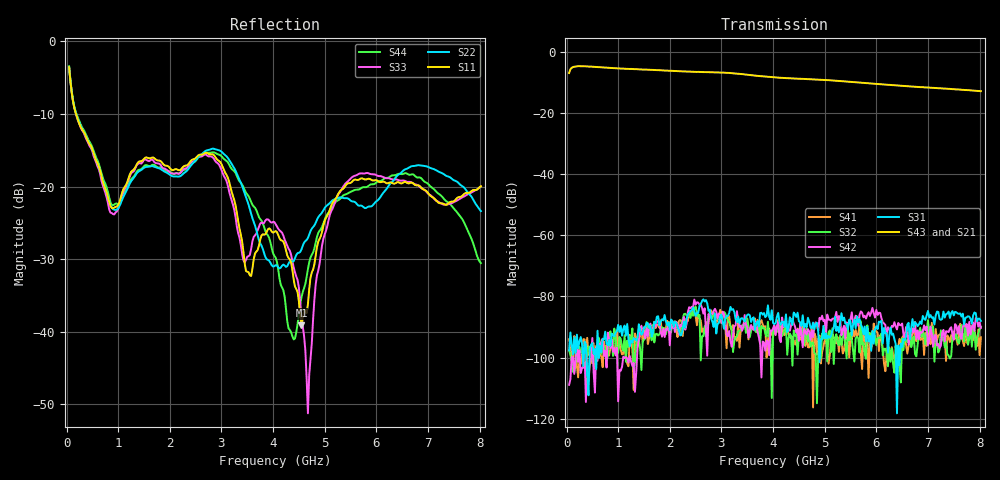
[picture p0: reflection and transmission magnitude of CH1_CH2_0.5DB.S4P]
!Agilent Technologies,E5071C,MY46316741,A.11.02
!Date: Thu May 28 14:25:22 2026
!Data & Calibration Information:
!1:CH1 INPUT 2:CH1 OUTPUT 3:CH2 INPUT 4:CH2 OUTPUT
!Freq	S11:SOLT4(ON)	S12:SOLT4(ON)	S13:SOLT4(ON)	S14:SOLT4(ON)
!	S21:SOLT4(ON)	S22:SOLT4(ON)	S23:SOLT4(ON)	S24:SOLT4(ON)
!	S31:SOLT4(ON)	S32:SOLT4(ON)	S33:SOLT4(ON)	S34:SOLT4(ON)
!	S41:SOLT4(ON)	S42:SOLT4(ON)	S43:SOLT4(ON)	S44:SOLT4(ON)
!PortZ  Port1:50+j0  Port2:50+j0  Port3:50+j0  Port4:50+j0
!Above PortZ is port z conversion or system Z0 setting when saving the data.
!When reading, reference impedance value at option line is always used.
# Hz S dB R 50
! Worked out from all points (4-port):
!   320 points, 50 MHz to 8.025 GHz, reference 50 ohm
!   strongest paths, dB at 50 MHz, 2.05 GHz, 4.05 GHz, 6.05 GHz, 8.025 GHz:
!     S43: -6.9, -6.2, -8.4, -10.5, -12.8
!     S21: -7.0, -6.3, -8.4, -10.5, -12.9
!     S31: -97.7, -88.0, -88.7, -88.2, -88.0
!     S42: -108.9, -90.3, -92.6, -85.3, -90.3
!     S32: -97.7, -88.7, -90.1, -93.5, -89.9
!     S41: -94.0, -89.4, -90.8, -97.8, -93.4
!   lowest |S11| = -39.1 dB at 4.55 GHz (marker M1), VSWR 1.02, Z = 49.7 - j1.05 ohm
!   |S11| at or under -10 dB: 183.6 MHz to end of sweep
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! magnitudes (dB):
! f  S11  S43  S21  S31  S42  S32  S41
! 50 MHz  -3.6  -6.9  -7.0  -97.7  -108.9  -97.7  -94.0
! 900 MHz  -23.0  -5.3  -5.4  -92.8  -98.1  -99.5  -94.0
! 2.85 GHz  -15.6  -6.7  -6.8  -90.0  -84.8  -85.1  -85.8
! 4.55 GHz  -39.1  -8.8  -8.9  -89.7  -92.5  -92.9  -94.2
! 4.675 GHz  -36.2  -8.9  -9.0  -87.0  -90.7  -94.8  -96.6
! 5.425 GHz  -19.7  -9.7  -9.7  -88.9  -88.5  -100.3  -94.1
! 8.025 GHz  -20.0  -12.8  -12.9  -88.0  -90.3  -89.9  -93.4
